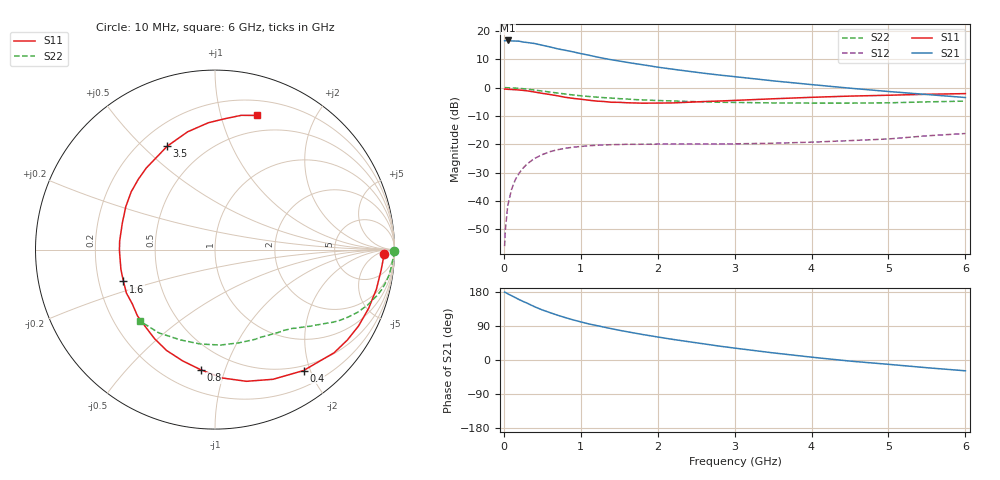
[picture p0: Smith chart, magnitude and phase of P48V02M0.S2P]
! SIEMENS Small Signal Semiconductors
! BFP182
! Si NPN RF Bipolar Junction Transistor in SOT143
! VCE = 8 V  IC = 2 mA
! Common Emitter S-Parameters:  March  1996
# GHz  S  MA  R  50
!  f  S11  S21  S12  S22
! GHz  MAG  ANG  MAG  ANG  MAG  ANG  MAG  ANG
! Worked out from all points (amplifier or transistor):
!   36 points, 10 MHz to 6 GHz, reference 50 ohm
!   highest |S21| = 16.6 dB at 50 MHz (marker M1)
!   |S21| within 3 dB of that: start of sweep to 709.2 MHz
!   unconditionally stable (mu >= 1): 2.255 GHz to end of sweep
!   at 250 MHz: K = 0.13, MSG = 22.2 dB, |S12| = -28.4 dB
!   at 1.4 GHz: K = 0.66, MSG = 15.0 dB, |S12| = -20.1 dB
!   at 6 GHz: K = 1.01, MAG = 5.8 dB, |S12| = -16.2 dB
!   lowest NFmin = 1.10 dB at 450 MHz
!   S11 on the Smith chart (normalised r, x): 10 MHz: 28, -11; 400 MHz: 0.43, -1.90; 800 MHz: 0.34, -0.83; 1.6 GHz: 0.31, -0.15; 3.5 GHz: 0.31, +0.60; 6 GHz: 0.34, +1.30
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0.01  0.9402 -1.4  6.704 179.1  0.0016 88.3  0.9952 -0.5
0.02  0.9404 -2.6  6.727 178.4  0.0031 84.5  0.9975 -1.1
0.05  0.9325 -7.1  6.775 174.7  0.0082 86.1  0.9936 -2.7
0.1  0.9259 -13.8  6.654 169.8  0.016 80.6  0.9873 -5.5
0.2  0.9059 -28.0  6.576 159.3  0.0311 73.7  0.9692 -10.8
0.3  0.8779 -40.9  6.246 150.3  0.0448 66.1  0.9405 -15.6
0.4  0.835 -53.8  5.982 140.5  0.0565 59.5  0.9052 -19.9
0.5  0.7916 -65.9  5.58 132.1  0.0658 52.7  0.8683 -23.7
0.6  0.7543 -76.6  5.208 125.0  0.0742 47.7  0.8337 -26.7
0.7  0.7158 -87.0  4.823 118.1  0.0803 43.0  0.8012 -29.4
0.8  0.674 -96.8  4.542 111.8  0.0851 38.8  0.7707 -31.7
0.9  0.6457 -106.2  4.269 105.9  0.089 35.4  0.7407 -33.7
1.1  0.6 -124.1  3.737 95.4  0.0944 29.6  0.6972 -37.2
1.3  0.5683 -139.5  3.274 86.8  0.0975 24.8  0.6647 -40.2
1.6  0.54 -160.8  2.786 74.7  0.1001 20.0  0.6284 -44.2
1.8  0.5314 -174.4  2.53 67.4  0.1003 18.2  0.607 -46.8
2.2  0.5369 164.2  2.105 54.3  0.1009 15.2  0.581 -52.6
2.8  0.5797 137.5  1.665 36.7  0.1014 13.8  0.5513 -62.2
3.5  0.6347 114.8  1.315 18.8  0.1044 14.3  0.5363 -75.6
4.5  0.7077 93.0  0.976 -2.9  0.1162 16.4  0.5324 -98.8
5.5  0.7624 78.9  0.755 -20.4  0.1412 17.3  0.5597 -124.0
6  0.7828 72.7  0.668 -28.5  0.155 14.6  0.5774 -136.5
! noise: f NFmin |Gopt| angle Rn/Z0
0.45  1.1  0.42  29  0.36
0.9  1.2  0.4  58  0.3
1.8  1.85  0.32  126  0.22
